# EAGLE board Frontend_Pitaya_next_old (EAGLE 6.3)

Size 60 x 105.71 mm. Coordinates in mm from the lower left corner, seen from the top.
Outline: 0,0 60,0 60,100.16 arc42 0,100.16 0,0
Copper layers (1*16): Top 0.035mm / dielectric 1.5mm / Bottom 0.035mm
Design rules "default": minimum track width 10mil, minimum drill 24mil, track to track 8mil, track to pad 8mil, pad to pad 8mil, via to via 8mil, smd to smd 8mil, copper to edge 40mil, drill to drill 8mil, minimum pad ring 10mil, minimum via ring 8mil, stop-mask expansion 4mil, vias tented up to drill 0mil, thermal gap 10mil
Holes 3.2 mm at 1.91,98.42 57.78,98.42 1.91,12.06 57.78,12.06

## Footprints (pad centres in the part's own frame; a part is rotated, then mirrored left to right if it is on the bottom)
C0805 = smd 1.3 x 1.5: 1 -0.85,0; 2 0.85,0
FE13-2 = drill 0.914: 1 -15.24,1.27 | drill 0.914 octagon: 2 -15.24,-1.27; 3 -12.7,1.27; 4 -12.7,-1.27; 5 -10.16,1.27; 6 -10.16,-1.27; 7 -7.62,1.27; 8 -7.62,-1.27; 9 -5.08,1.27; 10 -5.08,-1.27; 11 -2.54,1.27; 12 -2.54,-1.27; 13 0,1.27; 14 0,-1.27; 15 2.54,1.27; 16 2.54,-1.27; 17 5.08,1.27; 18 5.08,-1.27; 19 7.62,1.27; 20 7.62,-1.27; 21 10.16,1.27; 22 10.16,-1.27; 23 12.7,1.27; 24 12.7,-1.27; 25 15.24,1.27; 26 15.24,-1.27
D2PACK = smd 2.083 x 3.81: 1 -2.54,-8.89; 3 2.54,-8.89 | smd 11.43 x 8.89: 2 0,2.54
R0805 = smd 1.3 x 1.5: 1 -0.85,0; 2 0.85,0
JAE_NEXT = smd 0.813 x 0.406: 3V3 -1.905,1.155; 5VA -1.905,2.755; 5VB -1.905,1.955; A+ 1.495,-1.245; A- 1.495,-0.445; CV+ 1.495,-3.645; CV- 1.495,-2.845; G1 1.495,2.755; G3 1.495,1.955; G5 1.495,1.155; G7 1.495,0.355; G8 -1.905,0.355; G13 1.495,-2.045; G14 -1.905,-2.045; G19 1.495,-4.445; G20 -1.905,-4.445; SC+ -1.905,-3.645; SC- -1.905,-2.845; SD+ -1.905,-1.245; SD- -1.905,-0.445 | hole 0.8: -0.205,3.455 | hole 1: -0.205,-5.045
MOLEX87833NEXT = drill 0.9: P$1 -1.27,1.27; P$2 -1.27,3.27; P$3 0.73,1.27; P$4 0.73,3.27; P$5 2.73,1.27; P$6 2.73,3.27; P$7 4.73,1.27; P$8 4.73,3.27
SN65LVDS104 = smd 1.524 x 0.635: P$1 -3.81,5.08; P$2 -3.81,3.81; P$3 -3.81,2.54; P$4 -3.81,1.27; P$5 -3.81,0; P$6 -3.81,-1.27; P$7 -3.81,-2.54; P$8 -3.81,-3.81; P$9 2.54,-3.81; P$10 2.54,-2.54; P$11 2.54,-1.27; P$12 2.54,0; P$13 2.54,1.27; P$14 2.54,2.54; P$15 2.54,3.81; P$16 2.54,5.08

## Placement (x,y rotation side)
C1  [C0805]  11.43,43.18 90 bottom
C2  [C0805]  43.18,55.88 270 bottom
E1  [FE13-2]  3.81,80.01 90 bottom
E2  [FE13-2]  55.88,80.01 90 bottom
E2_EXT  [FE13-2]  55.88,34.29 90 bottom
IC2  LD117AD2MTR  [D2PACK]  44.45,36.83 180 bottom
R1  150  [R0805]  2.54,41.91 270 bottom
R2  150  [R0805]  6.35,48.26 270 bottom
R3  150  [R0805]  6.35,41.91 270 bottom
R4  150  [R0805]  2.54,48.26 270 bottom
R5  100  [R0805]  12.7,48.26 90 bottom
U$1  JAE_NEXT  [JAE_NEXT]  13.97,92.71 0 top
U$2  MOLEX87833_NEXT  [MOLEX87833NEXT]  11.43,17.78 270 top
U$3  SN65LVDS104  [SN65LVDS104]  29.21,54.61 0 bottom
U$4  MOLEX87833_NEXT  [MOLEX87833NEXT]  25.4,17.78 270 top
U$5  JAE_NEXT  [JAE_NEXT]  27.94,92.71 0 top
U$6  MOLEX87833_NEXT  [MOLEX87833NEXT]  39.37,17.78 270 top
U$7  JAE_NEXT  [JAE_NEXT]  41.91,92.71 0 top

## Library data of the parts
C1 C2 R1-R5 = resistor
E1 E2 E2_EXT = con-lsta; OC_FARNELL: unknown; OC_NEWARK: unknown
IC2 = v-reg
U$1 U$5 U$7 = JAE_next
U$2 U$4 U$6 = molex 87833 next
U$3 = SN65LVDS104

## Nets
+3V3: C1.1 IC2.2 R1.2 R3.2
GND: C1.2 IC2.1 R2.1 R4.1
N$1: E2.1 E2_EXT.1
N$2: E2.3 E2_EXT.3
N$3: E2.5 E2_EXT.5
N$4: E2.2 E2_EXT.2
N$5: E2.4 E2_EXT.4
N$6: E2.6 E2_EXT.6
N$7: U$2.P$1 U$2.P$2 U$2.P$4 U$2.P$6 U$2.P$7 U$2.P$8
N$8: E2.7 E2_EXT.7
N$9: E2.9 E2_EXT.9
N$10: E2.8 E2_EXT.8
N$11: E2.10 E2_EXT.10
N$12: E2.11 E2_EXT.11
N$13: E2.13 E2_EXT.13
N$14: E2.15 E2_EXT.15
N$15: E2.12 E2_EXT.12
N$16: E2.14 E2_EXT.14
N$17: E2.16 E2_EXT.16
N$18: E2.17 E2_EXT.17
N$19: E2.19 E2_EXT.19
N$20: E2.18 E2_EXT.18
N$21: E2.20 E2_EXT.20
N$22: E2.21 E2_EXT.21
N$23: E2.23 E2_EXT.23
N$24: E2.25 E2_EXT.25
N$25: E2.22 E2_EXT.22
N$26: E2.24 E2_EXT.24
N$27: E2.26 E2_EXT.26
N$28: U$4.P$1 U$4.P$2 U$4.P$4 U$4.P$6 U$4.P$7 U$4.P$8
N$29: U$6.P$1 U$6.P$2 U$6.P$4 U$6.P$6 U$6.P$7 U$6.P$8
N$30: R1.1 R2.2 R5.2
N$31: R3.1 R4.2 R5.1
N$34: C2.1 U$3.P$4
N$35: C2.2 U$3.P$5
N$36: IC2.3

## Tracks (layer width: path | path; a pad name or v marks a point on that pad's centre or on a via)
+3V3  (3 unrouted)
GND  (3 unrouted)
N$1  (1 unrouted)
N$2  (1 unrouted)
N$3  (1 unrouted)
N$4  (1 unrouted)
N$5  (1 unrouted)
N$6  (1 unrouted)
N$7  (5 unrouted)
N$8  (1 unrouted)
N$9  (1 unrouted)
N$10  (1 unrouted)
N$11  (1 unrouted)
N$12  (1 unrouted)
N$13  (1 unrouted)
N$14  (1 unrouted)
N$15  (1 unrouted)
N$16  (1 unrouted)
N$17  (1 unrouted)
N$18  (1 unrouted)
N$19  (1 unrouted)
N$20  (1 unrouted)
N$21  (1 unrouted)
N$22  (1 unrouted)
N$23  (1 unrouted)
N$24  (1 unrouted)
N$25  (1 unrouted)
N$26  (1 unrouted)
N$27  (1 unrouted)
N$28  (5 unrouted)
N$29  (5 unrouted)
N$30  (2 unrouted)
N$31  (2 unrouted)
N$34  (1 unrouted)
N$35  (1 unrouted)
